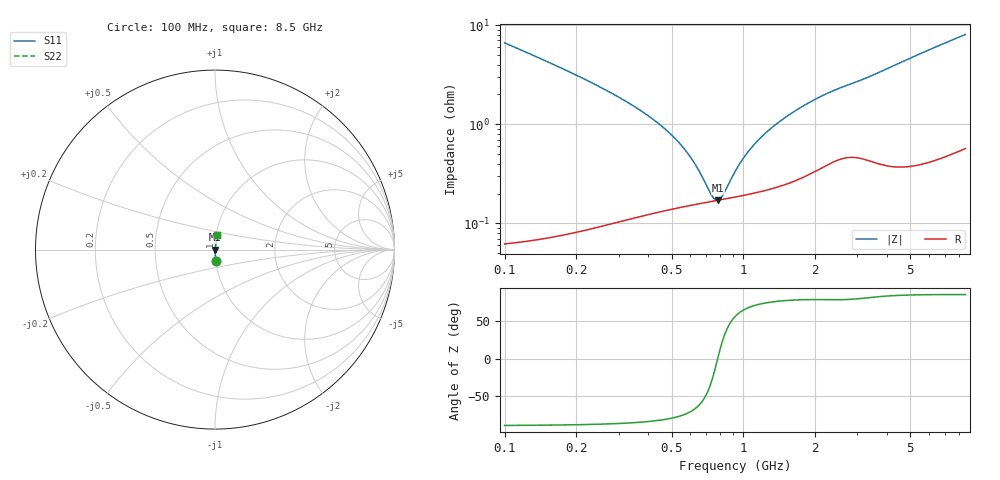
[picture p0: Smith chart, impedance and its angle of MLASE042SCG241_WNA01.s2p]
! MLASE042SCG241_WNA01  S-PARAMETER MODEL  ( General Type )
! Model Generated by TAIYO YUDEN Corporation (http://www.ty-top.com)
! Version 1.0
! TAIYO YUDEN Control No. 180301
! Copyright(c) 2018 TAIYO YUDEN CO.,LTD. All Rights Reserved.
! Product Description (link to TY-COMPAS)
! https://ds.yuden.co.jp/TYCOMPAS/or/detail?pn=MLASE042SCG241JWNA01&u=M
! Products Name : Multilayer Ceramic Capacitors
! Characteristics :
!  Capacitance : 240 pF , Rated Voltage : 16V , TCC : CG / C0G
!  Case Size : 0.4 x 0.2 / 0.016 x 0.008 [mm/inch] , Thickness : 0.2 / 0.008 [mm/inch]
!  (Conditions: Temperature = 25 degC , DC Bias Current/Voltage = 0A / 0V)
! External Node Assignments :
!  1  o---| |---o  2
! GND o---------o GND
! Frequency Range : 100MHz  -  8500MHz  [ 401 STEP ]
# MHz S RI R 50
! Freq[MHz].  S11 Real  S11 Imag  S21 Real  S21 Imag  S12 Real  S12 Imag  S22 Real  S22 Imag
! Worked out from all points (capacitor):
!   401 points, 100 MHz to 8.5 GHz, reference 50 ohm
!   read as one part in series: C = 237 pF near 102.2 MHz
!   lowest |Z| = 171 mohm at 780.5 MHz (marker M1)
!   series resonance near 780.1 MHz, so ESL is about 180 pH
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100  0.00498 -0.0658  0.995 0.0658  0.995 0.0658  0.00498 -0.0658
154.2121  0.00246 -0.0416  0.9975 0.0416  0.9975 0.0416  0.00246 -0.0416
224.9671  0.0016 -0.0271  0.9984 0.0271  0.9984 0.0271  0.0016 -0.0271
535.0023  0.00148 -0.00642  0.9985 0.00642  0.9985 0.00642  0.00148 -0.00642
618.1043  0.00155 -0.00389  0.9984 0.00389  0.9984 0.00389  0.00155 -0.00389
730.1548  0.00166 -0.00109  0.9983 0.00109  0.9983 0.00109  0.00166 -0.00109
754.8934  0.00168 -0.000542  0.9983 0.000542  0.9983 0.000542  0.00168 -0.000542
780.4701  0.00171 7.53e-06  0.9983 -7.53e-06  0.9983 -7.53e-06  0.00171 7.53e-06
815.9254  0.00174 0.000739  0.9983 -0.000739  0.9983 -0.000739  0.00174 0.000739
901.7006  0.00183 0.00239  0.9982 -0.00239  0.9982 -0.00239  0.00183 0.00239
963.8371  0.00189 0.0035  0.9981 -0.0035  0.9981 -0.0035  0.00189 0.0035
1077.058  0.00201 0.00538  0.998 -0.00538  0.998 -0.00538  0.00201 0.00538
1258.255  0.00224 0.00812  0.9978 -0.00812  0.9978 -0.00812  0.00224 0.00812
1502.954  0.0026 0.0115  0.9974 -0.0115  0.9974 -0.0115  0.0026 0.0115
1775.41  0.00312 0.0149  0.9969 -0.0149  0.9969 -0.0149  0.00312 0.0149
2097.259  0.00389 0.0185  0.9961 -0.0185  0.9961 -0.0185  0.00389 0.0185
2450.088  0.00475 0.0218  0.9952 -0.0218  0.9952 -0.0218  0.00475 0.0218
2926.566  0.00527 0.0258  0.9947 -0.0258  0.9947 -0.0258  0.00527 0.0258
4317.005  0.00523 0.039  0.9948 -0.039  0.9948 -0.039  0.00523 0.039
5762.285  0.00687 0.0533  0.9931 -0.0533  0.9931 -0.0533  0.00687 0.0533
7116.102  0.00916 0.0662  0.9908 -0.0662  0.9908 -0.0662  0.00916 0.0662
8500  0.0119 0.0788  0.9881 -0.0788  0.9881 -0.0788  0.0119 0.0788
